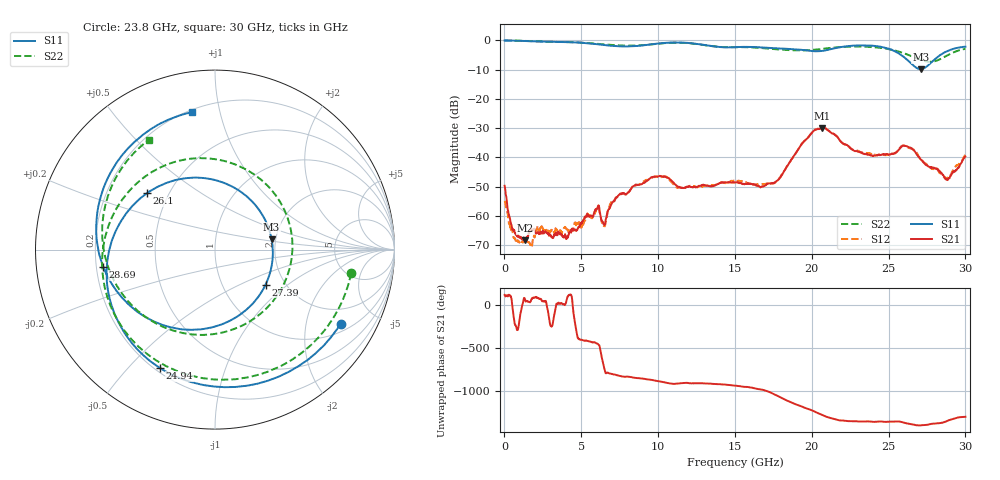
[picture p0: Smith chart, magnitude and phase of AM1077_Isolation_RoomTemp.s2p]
# Hz S DB R 50.0
!freq dBS11 angS11 dBS21 angS21 dBS12 angS12 dBS22 angS22
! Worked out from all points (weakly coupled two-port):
!   1601 points, 10 MHz to 30 GHz, reference 50 ohm
!   highest |S21| = -29.95 dB at 20.68 GHz (marker M1); lowest = -68.3 dB at 1.36 GHz (marker M2)
!   lowest |S11| = -9.9 dB at 27.09 GHz (marker M3), VSWR 1.94, Z = 95.1 + j11.9 ohm
!   |S11| at or under -10 dB: nowhere
!   |S22| runs from -7.4 to -0.1 dB; largest |S21 - S12| = 0.0049
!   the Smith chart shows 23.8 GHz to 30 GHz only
!   S11 on the Smith chart (normalised r, x): 23.8 GHz: 1.31, -3.17; 24.94 GHz: 0.22, -0.61; 26.1 GHz: 0.38, +0.31; 27.39 GHz: 1.59, -0.70; 28.69 GHz: 0.23, -0.07; 30 GHz: 0.21, +0.83
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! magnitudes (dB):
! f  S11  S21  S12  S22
! 10 MHz  -0.1  -49.7  -55.0  -0.1
! 572.3 MHz  -0.1  -64.7  -66.8  -0.1
! 1.36 GHz  -0.2  -68.3  -68.3  -0.2
! 4.002 GHz  -0.6  -67.8  -64.3  -0.6
! 5.015 GHz  -0.8  -62.8  -64.1  -0.8
! 6.045 GHz  -1.3  -57.4  -57.1  -1.2
! 6.477 GHz  -1.6  -63.0  -63.5  -1.4
! 7.414 GHz  -2.0  -53.1  -53.2  -1.7
! 10.02 GHz  -1.1  -46.6  -46.8  -1.2
! 11.37 GHz  -0.8  -50.1  -50.4  -0.8
! 15.01 GHz  -2.4  -48.5  -48.0  -2.4
! 17.67 GHz  -2.7  -48.3  -48.4  -3.1
! 20.01 GHz  -3.7  -31.6  -31.6  -3.3
! 20.68 GHz  -3.6  -30.0  -30.0  -3.0
! 23.8 GHz  -1.8  -39.2  -38.8  -2.3
! 24.94 GHz  -2.8  -38.9  -39.2  -2.9
! 25.01 GHz  -2.9  -39.1  -39.2  -3.0
! 26.1 GHz  -6.1  -36.2  -36.3  -4.6
! 27.09 GHz  -9.9  -40.7  -40.7  -6.7
! 27.39 GHz  -9.3  -42.5  -42.1  -7.2
! 28.69 GHz  -4.0  -47.4  -47.0  -5.5
! 30 GHz  -2.2  -39.7  -39.2  -2.9
